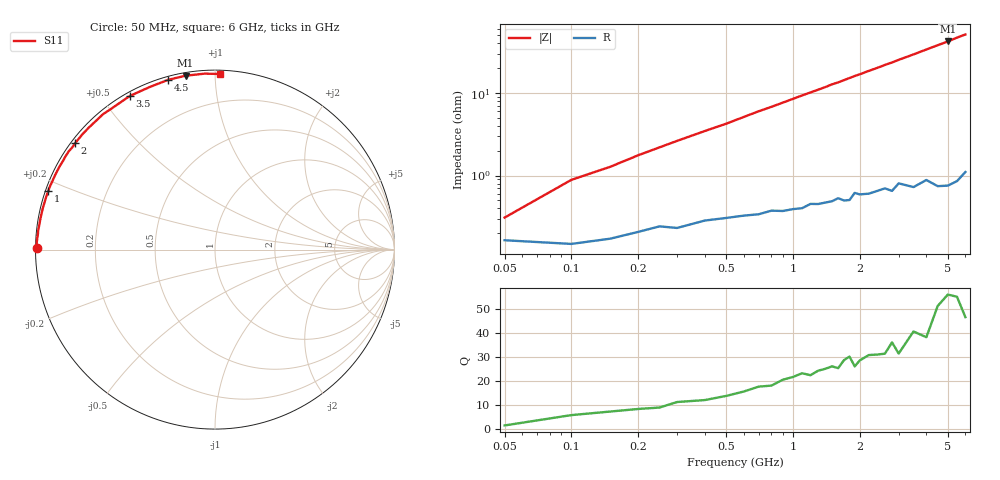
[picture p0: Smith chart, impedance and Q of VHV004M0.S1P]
! Infineon Technologies  Discrete & RF Semiconductors
! BB 814
! Si Tuning Diode in SOT23
! VR =
! S-Parameters:  July  1999
# GHz  S  MA  R  50
!  f  S11
! GHz  MAG  ANG
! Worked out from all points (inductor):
!   34 points, 50 MHz to 6 GHz, reference 50 ohm
!   read as one part to ground: L = 1.39 nH near 100 MHz
!   highest Q = 55.1 at 5 GHz (marker M1), where L = 1.34 nH
!   S11 on the Smith chart (normalised r, x): 50 MHz: 0.00, +0.01; 1 GHz: 0.01, +0.17; 2 GHz: 0.01, +0.34; 3.5 GHz: 0.01, +0.59; 4.5 GHz: 0.01, +0.76; 6 GHz: 0.02, +1.03
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0.05  0.9935 179.4
0.1  0.9941 178.0
0.15  0.9932 177.1
0.3  0.9908 174.0
0.5  0.9879 170.3
0.6  0.9872 168.3
0.7  0.9867 166.3
0.8  0.9854 164.5
1  0.9849 160.7
1.1  0.9846 158.8
1.3  0.9829 155.2
1.5  0.9819 151.4
1.6  0.9804 149.8
1.7  0.9818 148.0
1.8  0.9817 146.1
1.9  0.9779 144.3
2  0.979 142.7
2.2  0.979 139.2
2.4  0.9779 136.0
2.6  0.9768 132.6
2.8  0.9789 129.6
3  0.9747 126.3
3.5  0.9787 119.0
4  0.976 111.9
4.5  0.9814 105.4
5  0.9826 99.6
5.5  0.982 93.4
6  0.9788 88.4
